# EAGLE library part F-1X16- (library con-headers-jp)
FEMALE HEADER
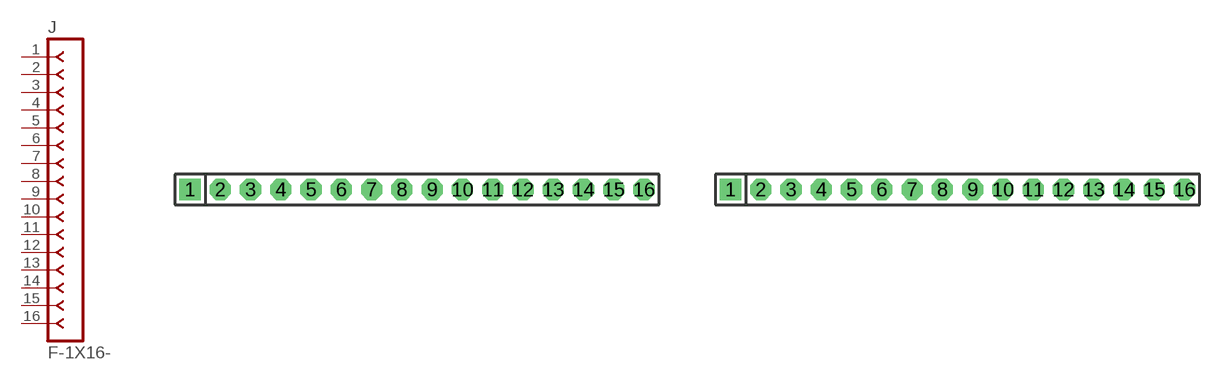
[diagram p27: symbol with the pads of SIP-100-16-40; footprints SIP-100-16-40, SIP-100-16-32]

Designator prefix J

## F-1X16-SIP-100-40  [SIP-100-16-40]
1  1  pas
2  2  pas
3  3  pas
4  4  pas
5  5  pas
6  6  pas
7  7  pas
8  8  pas
9  9  pas
10  10  pas
11  11  pas
12  12  pas
13  13  pas
14  14  pas
15  15  pas
16  16  pas

## F-1X16-SIP-100-32  [SIP-100-16-32]
Pads as for SIP-100-16-40

## F-1X16-SIP-100-32Y  [SIP-100-16-32Y]
Pads as for SIP-100-16-40

## F-1X16-SIP-100-40Y  [SIP-100-16-40Y]
Pads as for SIP-100-16-40

## F-1X16-KK-4455-B16  [KK-4455-B16]
Pads as for SIP-100-16-40

## F-1X16-KK-4455-C16  [KK-4455-C16]
Pads as for SIP-100-16-40

## F-1X16-KK-4455-A16  [KK-4455-A16]
Pads as for SIP-100-16-40

## Footprint SIP-100-16-40 (pad centres in mm)
SIP Header - 0.1", 40 mil drill
drill 1.016 pad 1.778 square: 1 -19.05,0
drill 1.016 pad 1.778 octagon: 2 -16.51,0; 3 -13.97,0; 4 -11.43,0; 5 -8.89,0; 6 -6.35,0; 7 -3.81,0; 8 -1.27,0; 9 1.27,0; 10 3.81,0; 11 6.35,0; 12 8.89,0; 13 11.43,0; 14 13.97,0; 15 16.51,0; 16 19.05,0

## Footprint SIP-100-16-32 (pad centres in mm)
SIP Header - 0.1", 32 mil drill
drill 0.813 pad 1.778 square: 1 -19.05,0
drill 0.813 pad 1.778 octagon: 2 -16.51,0; 3 -13.97,0; 4 -11.43,0; 5 -8.89,0; 6 -6.35,0; 7 -3.81,0; 8 -1.27,0; 9 1.27,0; 10 3.81,0; 11 6.35,0; 12 8.89,0; 13 11.43,0; 14 13.97,0; 15 16.51,0; 16 19.05,0

## Footprint SIP-100-16-32Y (pad centres in mm)
SIP Header - 0.1", 32 mil drill
drill 0.813 long: 1 -19.05,0; 2 -16.51,0; 3 -13.97,0; 4 -11.43,0; 5 -8.89,0; 6 -6.35,0; 7 -3.81,0; 8 -1.27,0; 9 1.27,0; 10 3.81,0; 11 6.35,0; 12 8.89,0; 13 11.43,0; 14 13.97,0; 15 16.51,0; 16 19.05,0

## Footprint SIP-100-16-40Y (pad centres in mm)
SIP Header - 0.1", 40 mil drill
drill 1.016 long: 1 -19.05,0; 2 -16.51,0; 3 -13.97,0; 4 -11.43,0; 5 -8.89,0; 6 -6.35,0; 7 -3.81,0; 8 -1.27,0; 9 1.27,0; 10 3.81,0; 11 6.35,0; 12 8.89,0; 13 11.43,0; 14 13.97,0; 15 16.51,0; 16 19.05,0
